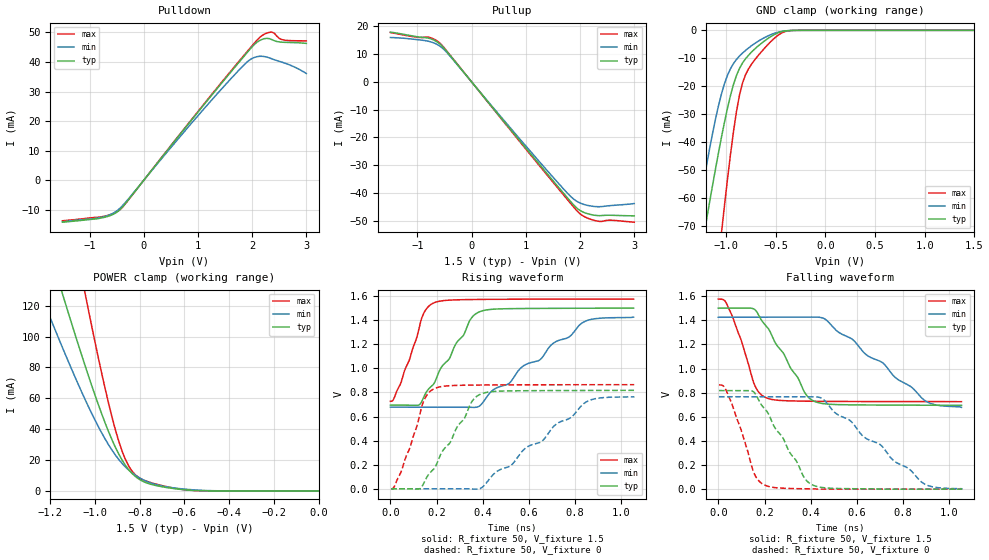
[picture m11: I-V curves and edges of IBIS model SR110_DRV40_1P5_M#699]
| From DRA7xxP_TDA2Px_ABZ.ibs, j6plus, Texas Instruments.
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| Model based on original model for DDR_DIFFIOPB_V
|   Sub model SR110_DRV40_1P5
[model]   SR110_DRV40_1P5_M#699
|[Description]  [1.5V-I/O-X-X]
|   , ,
|[Input Load]
|[Output Drive]
|Voltage   1.5V
|Mode   I/O
Model_type   I/O
Polarity   Non-Inverting
Enable   Active-Low
Vinl =  0.65
Vinh =  0.85
Cref =  15.0000pF
Rref =  100.0000M
Vref =  0V
Vmeas =  0.75
C_comp   2p   2p   2p
[Model Spec]
Vinl   0.65   0.6125   0.6875
Vinh   0.85   0.8125   0.8875
[Receiver Thresholds]
Tslew_ac = 0.5n
Vth = 0.75
Vth_max = 0.7875
Vth_min = 0.675
Vinh_ac = 0.175
Vinh_dc = 0.1
Vinl_ac = -0.175
Vinl_dc = -0.1
[Temperature Range]   25   125   -40
[Voltage Range]   1.5   1.425   1.575
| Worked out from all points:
|   slope of the pulldown table from 0 to 0.225 V, typ, clamps not added: 43 ohm
|   slope of the pullup table from 0 to 0.225 V, typ, clamps not added: 41.7 ohm
|   GND clamp passes 1 mA (typ) near -0.48 V on its own axis
|   POWER clamp passes 1 mA (typ) near -0.62 V on its own axis
|   rising waveform, R_fixture 50, V_fixture 1.5: 20-80 % time 150ps typ, 333ps min, 85.3ps max; typ from 0.695 V to 1.5 V
|   rising waveform, R_fixture 50, V_fixture 0: 20-80 % time 148ps typ, 325ps min, 85.2ps max; typ from 0 V to 0.817 V
|   falling waveform, R_fixture 50, V_fixture 1.5: 20-80 % time 147ps typ, 302ps min, 84.7ps max; typ from 1.5 V to 0.695 V
|   falling waveform, R_fixture 50, V_fixture 0: 20-80 % time 148ps typ, 313ps min, 85.3ps max; typ from 0.817 V to 0 V
[POWER_clamp]
-1.5V     302.8mA    223.9mA    484.4mA
-1.242V   174.3mA    127.3mA    279.1mA
-1.136V   123.3mA    89.68mA    196.8mA
-1.045V   81.65mA    59.62mA    128.8mA
-1.03V    75mA       54.92mA    117.8mA
-939.4mV  38.44mA    29.91mA    56.84mA
-893.9mV  23.93mA    20.41mA    32.31mA
-848.5mV  13.61mA    13.43mA    15.91mA
-803mV    7.623mA    8.663mA    8.564mA
-712.1mV  3.022mA    3.561mA    3.877mA
-575.8mV  470.5uA    872uA      449uA
0V        112.6nA    435.6nA    613.8nA
[Pulldown]
-1.5V     -14.18mA   -14.05mA   -13.7mA
-727.3mV  -12.54mA   -12.27mA   -12.15mA
-545.5mV  -11.35mA   -10.95mA   -11.1mA
-409.1mV  -9.378mA   -8.925mA   -9.416mA
1.227V    28.16mA    26.58mA    28.43mA
1.818V    41.23mA    38.42mA    41.56mA
2V        45.11mA    41.2mA     45.49mA
2.182V    47.62mA    41.92mA    48.94mA
2.273V    47.99mA    41.65mA    49.78mA
2.364V    47.57mA    41.06mA    50.1mA
2.545V    46.7mA     39.96mA    47.58mA
3V        46.28mA    36.09mA    47.12mA
[Pullup]
-1.5V     17.97mA    16.01mA    17.82mA
-1V       16.28mA    15.23mA    16.1mA
-772.7mV  15.66mA    14.54mA    16.02mA
-590.9mV  13.75mA    12.97mA    14.08mA
-409.1mV  9.799mA    9.534mA    9.955mA
1.409V    -33.42mA   -32.26mA   -33.94mA
1.773V    -41.87mA   -40.19mA   -42.52mA
1.909V    -44.87mA   -42.6mA    -45.68mA
2.091V    -47.15mA   -44.23mA   -48.65mA
2.318V    -48.13mA   -44.93mA   -50.11mA
2.591V    -48.02mA   -44.49mA   -49.82mA
3V        -48.22mA   -43.8mA    -50.51mA
[GND_clamp]
-1.5V     -133.6mA   -115.7mA   -234.3mA
-1.288V   -87.29mA   -67.59mA   -156.8mA
-1.197V   -68.11mA   -48.64mA   -124.4mA
-1.045V   -38.25mA   -22.77mA   -72.51mA
-1.015V   -32.88mA   -19.1mA    -62.74mA
-954.5mV  -23.3mA    -13.72mA   -44.4mA
-863.6mV  -13.6mA    -9.192mA   -23.11mA
-803mV    -10.18mA   -7.193mA   -15.89mA
-681.8mV  -5.771mA   -4.027mA   -9.287mA
-500mV    -1.264mA   -914.7uA   -2.429mA
-348.5mV  -52.39uA   -75.11uA   -85.87uA
1.5V      112.6nA    528.1nA    514.5nA
[Ramp]
dV/dt_f 0.48378155/0.14722271n 0.44934206/0.30342318n 0.51009285/84.796831p
dV/dt_r 0.49179862/0.14872035n 0.46157011/0.32678085n 0.51956908/85.385088p
R_load = 50
[Rising Waveform]
R_fixture = 50
V_fixture = 1.5
V_fixture_min = 1.425
V_fixture_max = 1.575
0s        694.7mV    677.7mV    726.3mV
44.52ps   694.1mV    677.6mV    874.2mV
124.4ps   696.9mV    677.6mV    1.336V
148.9ps   779.8mV    677.6mV    1.474V
189.2ps   875mV      677.7mV    1.544V
347ps     1.407V     676mV      1.571V
389ps     1.472V     692mV      1.572V
441.9ps   1.49V      816.2mV    1.573V
835.7ps   1.499V     1.384V     1.575V
1.053ns   1.5V       1.425V     1.575V
[Rising Waveform]
R_fixture = 50
V_fixture = 0
V_fixture_min = 0
V_fixture_max = 0
2.944ps   0V         0V         0V
47.15ps   0V         0V         144.9mV
128.2ps   0V         0V         625.5mV
153.9ps   82.68mV    0V         765.8mV
192.3ps   175.5mV    0V         833.4mV
351.3ps   719.5mV    -2.146mV   860.8mV
394ps     788.5mV    7.501mV    861.6mV
453.8ps   808.8mV    133.7mV    862.5mV
848ps     816.2mV    721.3mV    863.9mV
1.056ns   817.1mV    766.1mV    864.1mV
[Falling Waveform]
R_fixture = 50
V_fixture = 1.5
V_fixture_min = 1.425
V_fixture_max = 1.575
0s        1.5V       1.425V     1.575V
29.01ps   1.5V       1.425V     1.559V
59.23ps   1.5V       1.425V     1.441V
151.3ps   1.496V     1.425V     892.8mV
209.2ps   1.348V     1.425V     755.7mV
376.5ps   792.9mV    1.425V     729.2mV
418.7ps   725.6mV    1.427V     728.3mV
580.2ps   698.7mV    1.242V     726.4mV
898.9ps   695.7mV    728.7mV    725.5mV
1.053ns   694.7mV    677.7mV    725.4mV
[Falling Waveform]
R_fixture = 50
V_fixture = 0
V_fixture_min = 0
V_fixture_max = 0
2.944ps   817.1mV    766.1mV    864.1mV
26.19ps   817.2mV    766.1mV    846.3mV
56.26ps   817.2mV    766.1mV    720.1mV
147.2ps   812.3mV    766.2mV    171.3mV
202.7ps   662mV      766.1mV    32.09mV
372ps     95.68mV    766.2mV    3.127mV
413.5ps   30.15mV    766.2mV    2.178mV
454ps     12.58mV    745.2mV    0V
888ps     0V         47.65mV    0V
1.056ns   0V         0V         0V
